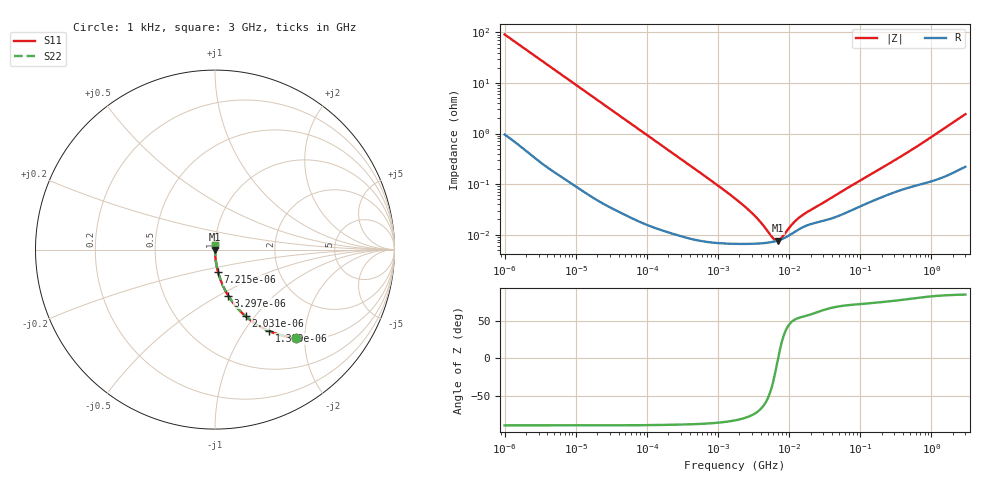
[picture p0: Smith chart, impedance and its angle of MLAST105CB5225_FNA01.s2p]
! MLAST105CB5225_FNA01  S-PARAMETER MODEL  ( Standard Model )
! Model Generated by TAIYO YUDEN Corporation (http://www.ty-top.com)
! Version 1.0
! TAIYO YUDEN Control No. 220601
! Copyright(c) 2013 TAIYO YUDEN CO.,LTD. All Rights Reserved.
! Product Description (link to TY-COMPAS)
! https://ds.yuden.co.jp/TYCOMPAS/or/detail?pn=MLAST105CB5225KFNA01&u=M
! Products Name : Multilayer Ceramic Capacitors
! Characteristics :
!  Capacitance : 2.2 [uF] , Rated Voltage : 25 [V] , TCC : X5R
!  Case Size : 1.0 x 0.5 / 0.039 x 0.02 [mm/inch] , Thickness : 0.5 / 0.02 [mm/inch]
!  (Conditions: Temperature = 25 [degC] , DC Bias Voltage = 0 [V])
! External Node Assignments :
!  1  o---| |---o  2
! GND o---------o GND
! Frequency Range : 1kHz  -  3GHz  [ 401 STEP ]
# MHZ S RI R 50
! Freq[MHz].  S11 Real  S11 Imag  S21 Real  S21 Imag  S12 Real  S12 Imag  S22 Real  S22 Imag
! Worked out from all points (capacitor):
!   401 points, 1 kHz to 3 GHz, reference 50 ohm
!   read as one part in series: C = 1.75 uF near 1.077 kHz
!   lowest |Z| = 7.62 mohm at 6.882 MHz (marker M1)
!   series resonance near 6.994 MHz, so ESL is about 300 pH
!   S11 on the Smith chart (normalised r, x): 1 kHz: 1.02, -1.82; 1.399 kHz: 1.01, -1.30; 2.031 kHz: 1.01, -0.90; 3.297 kHz: 1.01, -0.56; 7.215 kHz: 1.00, -0.26; 3 GHz: 1.00, +0.05
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0.001  0.453 -0.4926  0.547 0.4926  0.547 0.4926  0.453 -0.4926
0.001399  0.3001 -0.4531  0.6999 0.4531  0.6999 0.4531  0.3001 -0.4531
0.002031  0.1709 -0.3715  0.8291 0.3715  0.8291 0.3715  0.1709 -0.3715
0.003297  0.0738 -0.2568  0.9262 0.2568  0.9262 0.2568  0.0738 -0.2568
0.007215  0.0172 -0.1252  0.9828 0.1252  0.9828 0.1252  0.0172 -0.1252
0.01216  0.00647 -0.0754  0.9935 0.0754  0.9935 0.0754  0.00647 -0.0754
0.033275  0.0011 -0.0279  0.9989 0.0279  0.9989 0.0279  0.0011 -0.0279
0.147855  0.000167 -0.00633  0.9998 0.00633  0.9998 0.00633  0.000167 -0.00633
0.734727  7.27e-05 -0.00128  0.9999 0.00128  0.9999 0.00128  7.27e-05 -0.00128
1.732051  6.6e-05 -0.000515  0.9999 0.000515  0.9999 0.000515  6.6e-05 -0.000515
3.264662  6.62e-05 -0.000228  0.9999 0.000228  0.9999 0.000228  6.62e-05 -0.000228
5.30084  7.01e-05 -7.67e-05  0.9999 7.67e-05  0.9999 7.67e-05  7.01e-05 -7.67e-05
5.711239  7.14e-05 -5.57e-05  0.9999 5.57e-05  0.9999 5.57e-05  7.14e-05 -5.57e-05
6.881678  7.61e-05 -4.37e-06  0.9999 4.37e-06  0.9999 4.37e-06  7.61e-05 -4.37e-06
7.988506  8.22e-05 3.61e-05  0.9999 -3.61e-05  0.9999 -3.61e-05  8.22e-05 3.61e-05
8.606987  8.62e-05 5.62e-05  0.9999 -5.62e-05  0.9999 -5.62e-05  8.62e-05 5.62e-05
12.97096  0.000122 0.000161  0.9999 -0.000161  0.9999 -0.000161  0.000122 0.000161
15.62917  0.000141 0.000203  0.9999 -0.000203  0.9999 -0.000203  0.000141 0.000203
21.06097  0.000165 0.000273  0.9998 -0.000273  0.9998 -0.000273  0.000165 0.000273
256.0921  0.000635 0.00248  0.9994 -0.00248  0.9994 -0.00248  0.000635 0.00248
650.4536  0.000988 0.00565  0.999 -0.00565  0.999 -0.00565  0.000988 0.00565
3000  0.00277 0.024  0.9972 -0.024  0.9972 -0.024  0.00277 0.024
